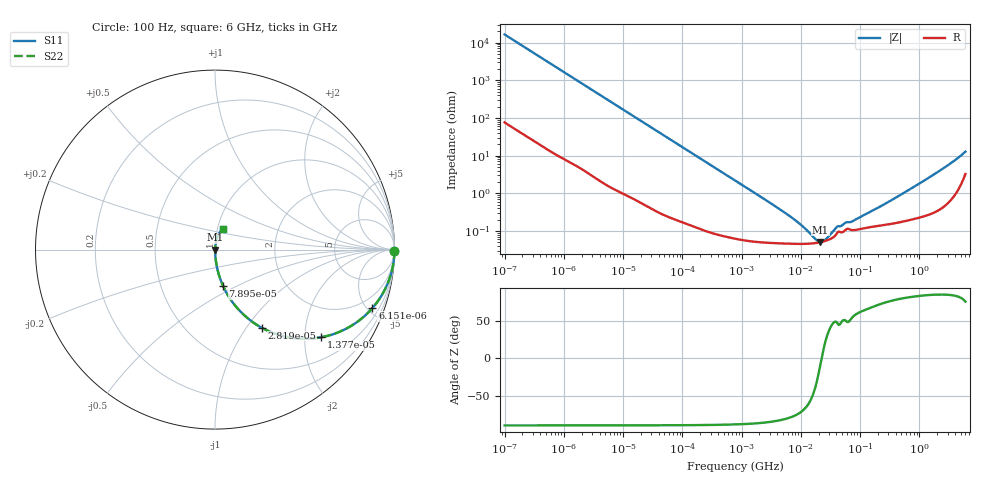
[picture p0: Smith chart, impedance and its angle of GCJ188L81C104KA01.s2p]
!Murata Part Number: GCJ188L81C104KA01
!These Parameters are Measured in Series Mode Connection
!Data Generated on Mar 13, 2026
!  o--ll--o
!Port1  Port2
!  o------o
!Operation Temp=25[degC], DC Bias Voltage=0[V]
!Freq. Start=100[Hz] Stop=6[GHz] 401[Steps]
# Hz S RI R 50
!Freq.(Hz) S11(Real) S11(Imag) S21(Real) S21(Imag) S12(Real) S12(Imag) S22(Real) S22(Imag)
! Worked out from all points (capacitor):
!   401 points, 100 Hz to 6 GHz, reference 50 ohm
!   read as one part in series: C = 97.2 nF near 109 Hz
!   lowest |Z| = 50.9 mohm at 21.28 MHz (marker M1)
!   series resonance near 22.52 MHz, so ESL is about 510 pH
!   S11 on the Smith chart (normalised r, x): 100 Hz: open; 6.151 kHz: 1.03, -5.38; 13.77 kHz: 1.02, -2.41; 28.19 kHz: 1.01, -1.18; 78.95 kHz: 1.00, -0.42; 6 GHz: 1.06, +0.25
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100  0.9999 -0.00612  6.59e-05 0.00612  6.59e-05 0.00612  0.9999 -0.00612
627  0.9984 -0.0381  0.00163 0.0381  0.00163 0.0381  0.9984 -0.0381
2008  0.9848 -0.1198  0.0152 0.1198  0.0152 0.1198  0.9848 -0.1198
6151  0.8773 -0.3255  0.1227 0.3255  0.1227 0.3255  0.8773 -0.3255
9204  0.7629 -0.4224  0.2371 0.4224  0.2371 0.4224  0.7629 -0.4224
13772  0.5916 -0.4884  0.4084 0.4884  0.4084 0.4884  0.5916 -0.4884
19704  0.4162 -0.4896  0.5838 0.4896  0.5838 0.4896  0.4162 -0.4896
28191  0.2599 -0.4351  0.7401 0.4351  0.7401 0.4351  0.2599 -0.4351
40335  0.1476 -0.3511  0.8524 0.3511  0.8524 0.3511  0.1476 -0.3511
78952  0.0445 -0.2018  0.9555 0.2018  0.9555 0.2018  0.0445 -0.2018
211427  0.00733 -0.0788  0.9927 0.0788  0.9927 0.0788  0.00733 -0.0788
774597  0.00109 -0.0218  0.9989 0.0218  0.9989 0.0218  0.00109 -0.0218
6353432  0.000463 -0.00248  0.9995 0.00248  0.9995 0.00248  0.000463 -0.00248
1.039699e7  0.000452 -0.00131  0.9995 0.00131  0.9995 0.00131  0.000452 -0.00131
1.555665e7  0.000465 -0.00058  0.9995 0.00058  0.9995 0.00058  0.000465 -0.00058
2.128304e7  0.000501 -8.61e-05  0.9995 8.61e-05  0.9995 8.61e-05  0.000501 -8.61e-05
2.545746e7  0.000538 0.000188  0.9995 -0.000188  0.9995 -0.000188  0.000538 0.000188
4.165952e7  0.000907 0.000952  0.9991 -0.000952  0.9991 -0.000952  0.000907 0.000952
7.797396e7  0.00105 0.00155  0.999 -0.00155  0.999 -0.00155  0.00105 0.00155
3.124326e8  0.00154 0.00586  0.9985 -0.00586  0.9985 -0.00586  0.00154 0.00586
1.791126e9  0.00406 0.0316  0.9959 -0.0316  0.9959 -0.0316  0.00406 0.0316
6e9  0.0447 0.1135  0.9553 -0.1135  0.9553 -0.1135  0.0447 0.1135
